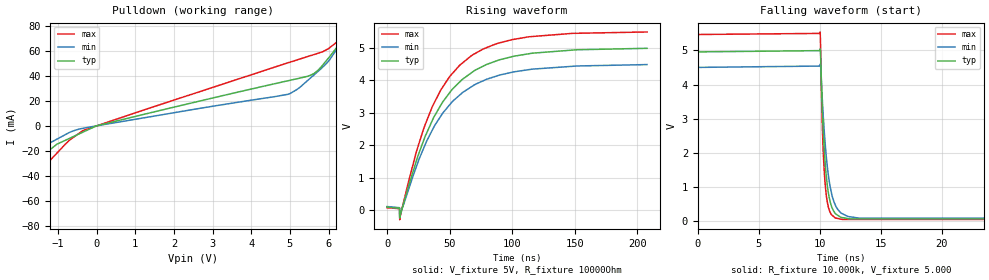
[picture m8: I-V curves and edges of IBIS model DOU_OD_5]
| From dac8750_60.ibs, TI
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[Model] DOU_OD_5  |5V opem drain digital output
Model_type   Open_drain
Polarity   Non-Inverting
Vmeas = 2.5
Vref = 2.5
Cref = 0pF
Rref = 10000
|   typ   min   max
|   (nom PVT)   (Fast PVT)   (slow PVT)
|   ON state : BUFFER OUTPUT TURNED HIGH
C_comp   1.722E-12   1.607E-12   1.837E-12
|   OFF state: BUFFER OUTPUT TURNED LOW
|C_comp   1.714E-12   1.585E-12   1.714E-12
| Where   nom PVT is  Nominal Process, 5.0V, 36C
|   Fast PVT is Strong Process, 5.5V, -40C
|   Slow PVT is Weak Process, 4.5V, 134C
|C_comp - from L-C Tank method, L = 1nH, peak frequency
[Voltage Range]   5   4.5   5.5
|Operating Temperature   27   125   -40
|Junction Temperature
[Temperature Range]   36   134   -40
[Pullup Reference]   5   4.5   5.5
[Pulldown Reference]   0   0   0
[Power Clamp Reference]   5   4.5   5.5
[GND Clamp Reference]   0   0   0
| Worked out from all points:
|   slope of the pulldown table from 0 to 0.75 V, typ, clamps not added: 133 ohm
|   falling waveform, R_fixture 10.000k, V_fixture 5.000: 20-80 % time 479ps typ, 679ps min, 326ps max; typ from 4.95 V to 0.065 V
|   rising waveform, V_fixture 5V, R_fixture 10000Ohm: 20-80 % time 39.7ns typ, 39.8ns min, 37.7ns max; typ from 0.1 V to 4.99 V
[Pulldown]
|   Voltage   I(typ)   I(min)   I(max)
-5V       -685.4mA   -536.9mA   -823.5mA
-2.816V   -105.1mA   -86.09mA   -204.7mA
-2.628V   -87.62mA   -77.53mA   -154.1mA
-2.463V   -79.57mA   -70.06mA   -109.8mA
-2.309V   -72.03mA   -63.06mA   -90.41mA
-1.243V   -19.97mA   -14.71mA   -28.97mA
-365.2mV  -5.185mA   -2.031mA   -3.924mA
4.966V    36.14mA    25.35mA    50.51mA
5.62V     41.75mA    40.57mA    56.93mA
6.253V    64.3mA     63.2mA     68.32mA
6.937V    106.5mA    99.37mA    105.3mA
9.985V    700mA      666mA      716.5mA
[Ramp]
R_load = 10000
|   typ   min   max
dV/dt_r   2.93354/3.97497e-008   2.62195/3.97081e-008   3.24609/3.75624e-008
dV/dt_f   2.9326/4.78694e-010   2.62109/6.76383e-010   3.24524/3.25889e-010
[Falling Waveform]
R_fixture = 10.000k
V_fixture = 5.000
V_fixture_min = 4.500
V_fixture_max = 5.500
C_fixture = 0.000
|  time   V(typ)   V(min)   V(max)
0s        4.953V     4.5V       5.461V
10.03ns   5.025V     4.568V     5.535V
10.07ns   4.88V      4.552V     5.105V
10.17ns   3.699V     3.839V     3.344V
10.27ns   2.783V     3.184V     2.184V
10.53ns   1.353V     1.928V     793.3mV
10.77ns   717.8mV    1.206V     352.3mV
11.06ns   365.9mV    696.8mV    171mV
11.85ns   114.6mV    228.1mV    60.42mV
207.8ns   65.31mV    84.39mV    52.34mV
[Rising Waveform]
V_fixture = 5V
V_fixture_min = 4.5V
V_fixture_max = 5.5V
R_fixture = 10000Ohm
C_fixture = 0F
|   Time   V(typ)   V(min)   V(max)
0s        100.1mV    118.4mV    82.32mV
10ns      65.31mV    82mV       52.34mV
10.16ns   -227.9mV   -153.8mV   -286.7mV
23.12ns   1.482V     1.308V     1.755V
35.79ns   2.733V     2.442V     3.158V
49.98ns   3.618V     3.246V     4.115V
67.36ns   4.233V     3.803V     4.759V
87.38ns   4.601V     4.134V     5.129V
112.8ns   4.818V     4.33V      5.341V
207.8ns   4.989V     4.488V     5.492V
